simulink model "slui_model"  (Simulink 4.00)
settings: Solver=ode15s  StartTime=0.0  StopTime=inf  FixedStep=0.1  RelTol=1e-3
undefined symbols (not defined in the file or in its folder): slui

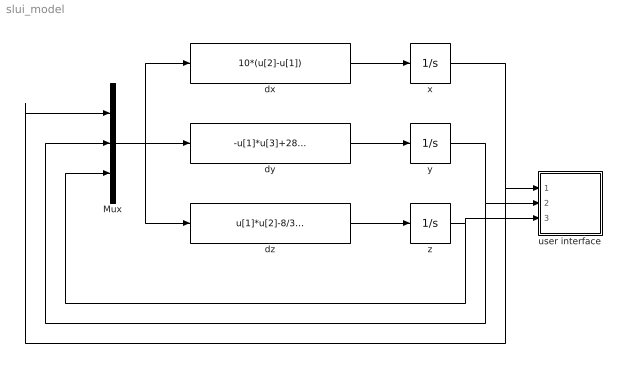
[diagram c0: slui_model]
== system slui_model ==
  Mux : Mux  Inputs=3
  dx : Fcn  Expr=10*(u[2]-u[1])
  dy : Fcn  Expr=-u[1]*u[3]+28*u[1]-u[2]
  dz : Fcn  Expr=u[1]*u[2]-8/3*u[3]
  user interface : Subsystem
  x : Integrator  ExternalReset=none  InitialConditionSource=internal  InitialCondition=5  LimitOutput=off  UpperSaturationLimit=inf  LowerSaturationLimit=-inf  ShowSaturationPort=off  ShowStatePort=off  AbsoluteTolerance=auto
  y : Integrator  ExternalReset=none  InitialConditionSource=internal  InitialCondition=-5  LimitOutput=off  UpperSaturationLimit=inf  LowerSaturationLimit=-inf  ShowSaturationPort=off  ShowStatePort=off  AbsoluteTolerance=auto
  z : Integrator  ExternalReset=none  InitialConditionSource=internal  InitialCondition=20  LimitOutput=off  UpperSaturationLimit=inf  LowerSaturationLimit=-inf  ShowSaturationPort=off  ShowStatePort=off  AbsoluteTolerance=auto
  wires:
  dy/1 -> y/1
  dz/1 -> z/1
  dx/1 -> x/1
  Mux/1 -> dz/1, dy/1, dx/1
  z/1 -> Mux/3, user interface/3(z)
  y/1 -> Mux/2, user interface/2(y)
  x/1 -> Mux/1, user interface/1(x)

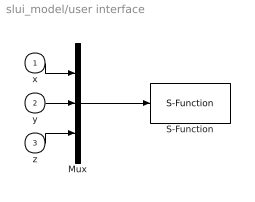
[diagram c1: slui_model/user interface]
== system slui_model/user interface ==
  x : Inport  Port=1  LatchInput=off
  y : Inport  Port=2  LatchInput=off
  z : Inport  Port=3  LatchInput=off
  Mux : Mux  Inputs=3
  S-Function : S-Function  LoadFcn=slui([], [], [], 'clear');  StartFcn=slui([], [], [], 'start');  StopFcn=slui([], [], [], 'stop');  FunctionName=slui  PortCounts=[]  SFunctionModules=''
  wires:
  Mux/1 -> S-Function/1
  x/1 -> Mux/1
  y/1 -> Mux/2
  z/1 -> Mux/3
